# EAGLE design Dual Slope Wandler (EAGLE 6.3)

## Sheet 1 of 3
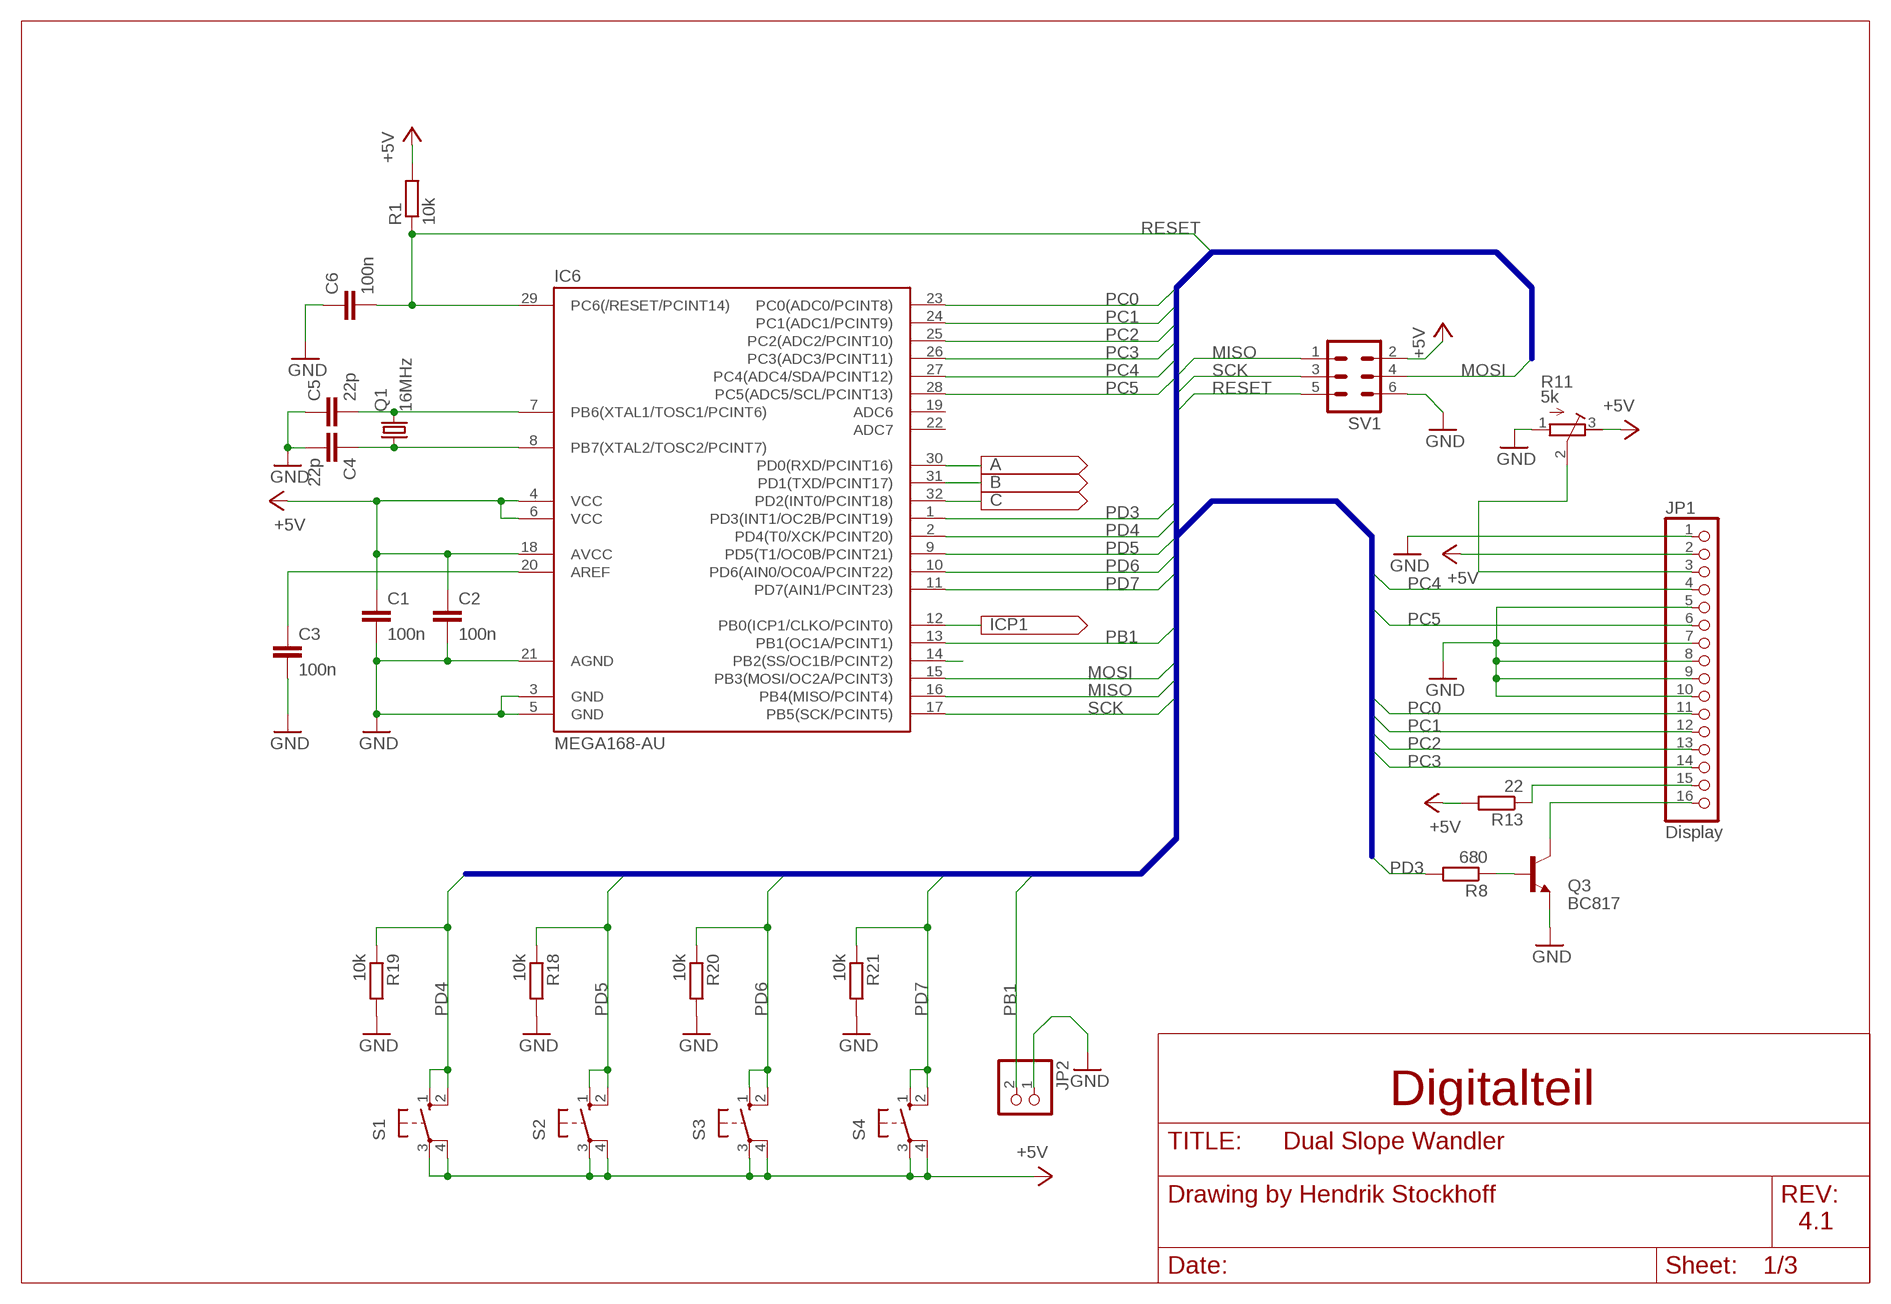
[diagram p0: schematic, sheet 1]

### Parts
C1  100n  C-EUC0805  [C0805]
C2  100n  C-EUC0805  [C0805]
C3  100n  C-EUC0805  [C0805]
C4  22p  C-EUC0805  [C0805]
C5  22p  C-EUC0805  [C0805]
C6  100n  C-EUC0805  [C0805]
IC6  MEGA168-AU  MEGA48/88/168-AU  [TQFP32-08]
JP1  Display  PINHD-1X16  [1X16]
JP2  PINHD-1X2  [1X02]
Q1  16MHz  CRYSTAL  [MT]
Q3  BC817  BC817-40SMD  [SOT23-BEC]
R1  10k  R-EU_R0805  [R0805]
R8  680  R-EU_R0805  [R0805]
R11  5k  R-TRIMM  [RTRIMC33X-2]
R13  22  R-EU_R0805  [R0805]
R18  10k  R-EU_R0805  [R0805]
R19  10k  R-EU_R0805  [R0805]
R20  10k  R-EU_R0805  [R0805]
R21  10k  R-EU_R0805  [R0805]
S1  10-XX  [B3F-10XX]
S2  10-XX  [B3F-10XX]
S3  10-XX  [B3F-10XX]
S4  10-XX  [B3F-10XX]
SV1  ML6  [ML6]

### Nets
+5V: C1.1 C2.1 IC6.4(VCC) IC6.6(VCC) IC6.18(AVCC) JP1.2 R1.2 R11.3(A) R13.2 S1.3(P) S1.4(P1) S2.3(P) S2.4(P1) S3.3(P) S3.4(P1) S4.3(P) S4.4(P1) SV1.2 ; also sheet 2,3
A: IC6.30(PD0(RXD/PCINT16)) ; also sheet 2
B: IC6.31(PD1(TXD/PCINT17)) ; also sheet 2
C: IC6.32(PD2(INT0/PCINT18)) ; also sheet 2
GND: C1.2 C2.2 C3.2 C4.2 C5.1 C6.1 IC6.3(GND) IC6.5(GND) IC6.21(AGND) JP1.1 JP1.5 JP1.7 JP1.8 JP1.9 JP1.10 JP2.1 Q3.E R11.1(E) R18.2 R19.2 R20.2 R21.2 SV1.6 ; also sheet 2,3
MISO: IC6.16(PB4(MISO/PCINT4)) SV1.1
MOSI: IC6.15(PB3(MOSI/OC2A/PCINT3)) SV1.4
N$4: JP1.3 R11.2(S)
N$6: C4.1 IC6.8(PB7(XTAL2/TOSC2/PCINT7)) Q1.1
N$7: C5.2 IC6.7(PB6(XTAL1/TOSC1/PCINT6)) Q1.3
N$15: IC6.14(PB2(SS/OC1B/PCINT2))
N$22: C3.1 IC6.20(AREF)
N$23: JP1.16 Q3.C
N$24: Q3.B R8.1
N$25: JP1.15 R13.1
PB0: IC6.12(PB0(ICP1/CLKO/PCINT0)) ; also sheet 2
PB1: IC6.13(PB1(OC1A/PCINT1)) JP2.2
PC0: IC6.23(PC0(ADC0/PCINT8)) JP1.11
PC1: IC6.24(PC1(ADC1/PCINT9)) JP1.12
PC2: IC6.25(PC2(ADC2/PCINT10)) JP1.13
PC3: IC6.26(PC3(ADC3/PCINT11)) JP1.14
PC4: IC6.27(PC4(ADC4/SDA/PCINT12)) JP1.4
PC5: IC6.28(PC5(ADC5/SCL/PCINT13)) JP1.6
PD3: IC6.1(PD3(INT1/OC2B/PCINT19)) R8.2
PD4: IC6.2(PD4(T0/XCK/PCINT20)) R19.1 S1.1(S) S1.2(S1)
PD5: IC6.9(PD5(T1/OC0B/PCINT21)) R18.1 S2.1(S) S2.2(S1)
PD6: IC6.10(PD6(AIN0/OC0A/PCINT22)) R20.1 S3.1(S) S3.2(S1)
PD7: IC6.11(PD7(AIN1/PCINT23)) R21.1 S4.1(S) S4.2(S1)
RESET: C6.2 IC6.29(PC6(/RESET/PCINT14)) R1.1 SV1.5
SCK: IC6.17(PB5(SCK/PCINT5)) SV1.3
Unconnected: IC6.19(ADC6) IC6.22(ADC7)

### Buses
MISO,MOSI,SCK,RESET,PC[0..5],PD[0..7],PB1

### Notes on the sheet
- Digitalteil
- 4.1

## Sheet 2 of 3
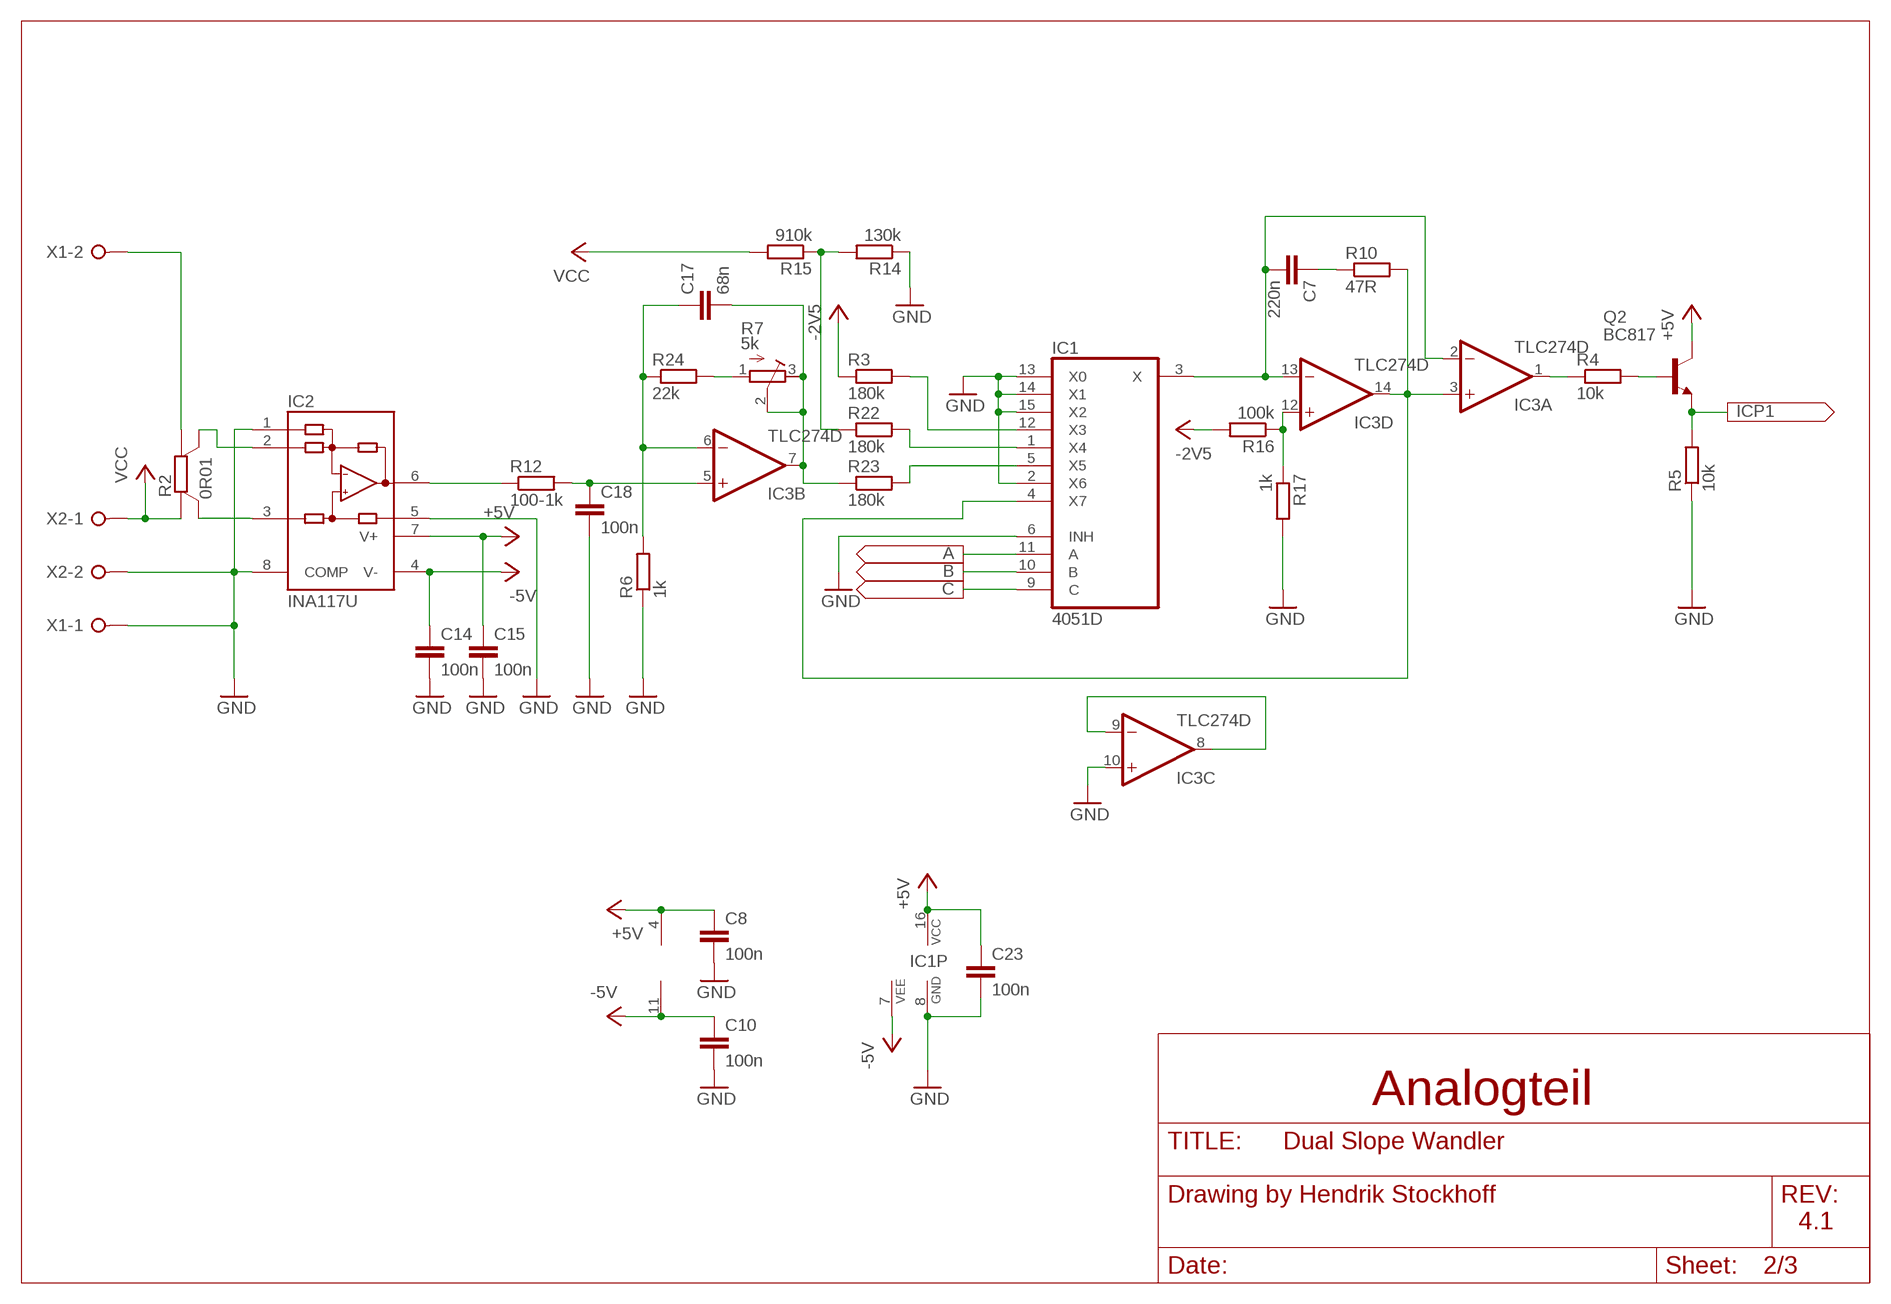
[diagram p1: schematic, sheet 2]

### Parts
C7  220n  C5/3  [C5B3]
C8  100n  C-EUC0805  [C0805]
C10  100n  C-EUC0805  [C0805]
C14  100n  C-EUC0805  [C0805]
C15  100n  C-EUC0805  [C0805]
C17  68n  C-EUC1206  [C1206]
C18  100n  C-EUC1206  [C1206]
C23  100n  C-EUC0805  [C0805]
IC1  4051D  [SO16]
IC2  INA117U  [SO08]
IC3  TLC274D  [SO14]
Q2  BC817  BC817-40SMD  [SOT23-BEC]
R2  0R01  PBV  [PBV]
R3  180k  R-EU_R0805  [R0805]
R4  10k  R-EU_R1206  [R1206]
R5  10k  R-EU_R1206  [R1206]
R6  1k  R-EU_R0805  [R0805]
R7  5k  R-TRIMM  [RTRIMC33X-2]
R10  47R  R-EU_R0805  [R0805]
R12  100-1k  R-EU_R0805  [R0805]
R14  130k  R-EU_R1206  [R1206]
R15  910k  R-EU_R1206  [R1206]
R16  100k  R-EU_R1206  [R1206]
R17  1k  R-EU_R1206  [R1206]
R22  180k  R-EU_R1206  [R1206]
R23  180k  R-EU_R0805  [R0805]
R24  22k  R-EU_R0805  [R0805]
X1  W237-02P  [W237-132]
X2  W237-02P  [W237-132]

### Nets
+5V: C8.1 C15.1 C23.1 IC1.16(VCC) IC2.7(V+) IC3.4(P:V+) Q2.C ; also sheet 1,3
-2V5: R3.1 R16.2 ; also sheet 3
-5V: C10.1 C14.1 IC1.7(VEE) IC2.4(V-) IC3.11(P:V-) ; also sheet 3
A: IC1.11(A) ; also sheet 1
B: IC1.10(B) ; also sheet 1
C: IC1.9(C) ; also sheet 1
GND: C8.2 C10.2 C14.2 C15.2 C18.2 C23.2 IC1.2(X6) IC1.6(INH) IC1.8(GND) IC1.13(X0) IC1.14(X1) IC1.15(X2) IC2.1(REFB) IC2.5(REFA) IC2.8(COMP) IC3.10(C:+IN) R5.1 R6.1 R14.1 R17.2 X1.1 X2.2 ; also sheet 1,3
N$5: C7.1 R10.1
N$8: IC2.6(OUT) R12.1
N$9: R2.I1(A) X1.2
N$10: IC1.4(X7) IC3.3(A:+IN) IC3.14(D:OUT) R10.2
N$11: IC3.8(C:OUT) IC3.9(C:-IN)
N$12: IC3.1(A:OUT) R4.1
N$13: Q2.B R4.2
N$14: IC1.5(X5) R23.2
N$16: R14.2 R15.1 R22.1
N$17: IC2.3(+IN) R2.U2(SB)
N$18: C18.1 IC3.5(B:+IN) R12.2
N$20: IC2.2(-IN) R2.U1(SA)
N$26: C17.2 IC3.7(B:OUT) R7.2(S) R7.3(A) R23.1
N$27: IC3.12(D:+IN) R16.1 R17.1
N$28: IC1.1(X4) R22.2
N$29: IC1.12(X3) R3.2
N$30: C7.2 IC1.3(X) IC3.2(A:-IN) IC3.13(D:-IN)
N$33: C17.1 IC3.6(B:-IN) R6.2 R24.1
N$35: R7.1(E) R24.2
PB0: Q2.E R5.2 ; also sheet 1
VCC: R2.I2(B) R15.2 X2.1 ; also sheet 3

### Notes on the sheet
- Analogteil
- 4.1

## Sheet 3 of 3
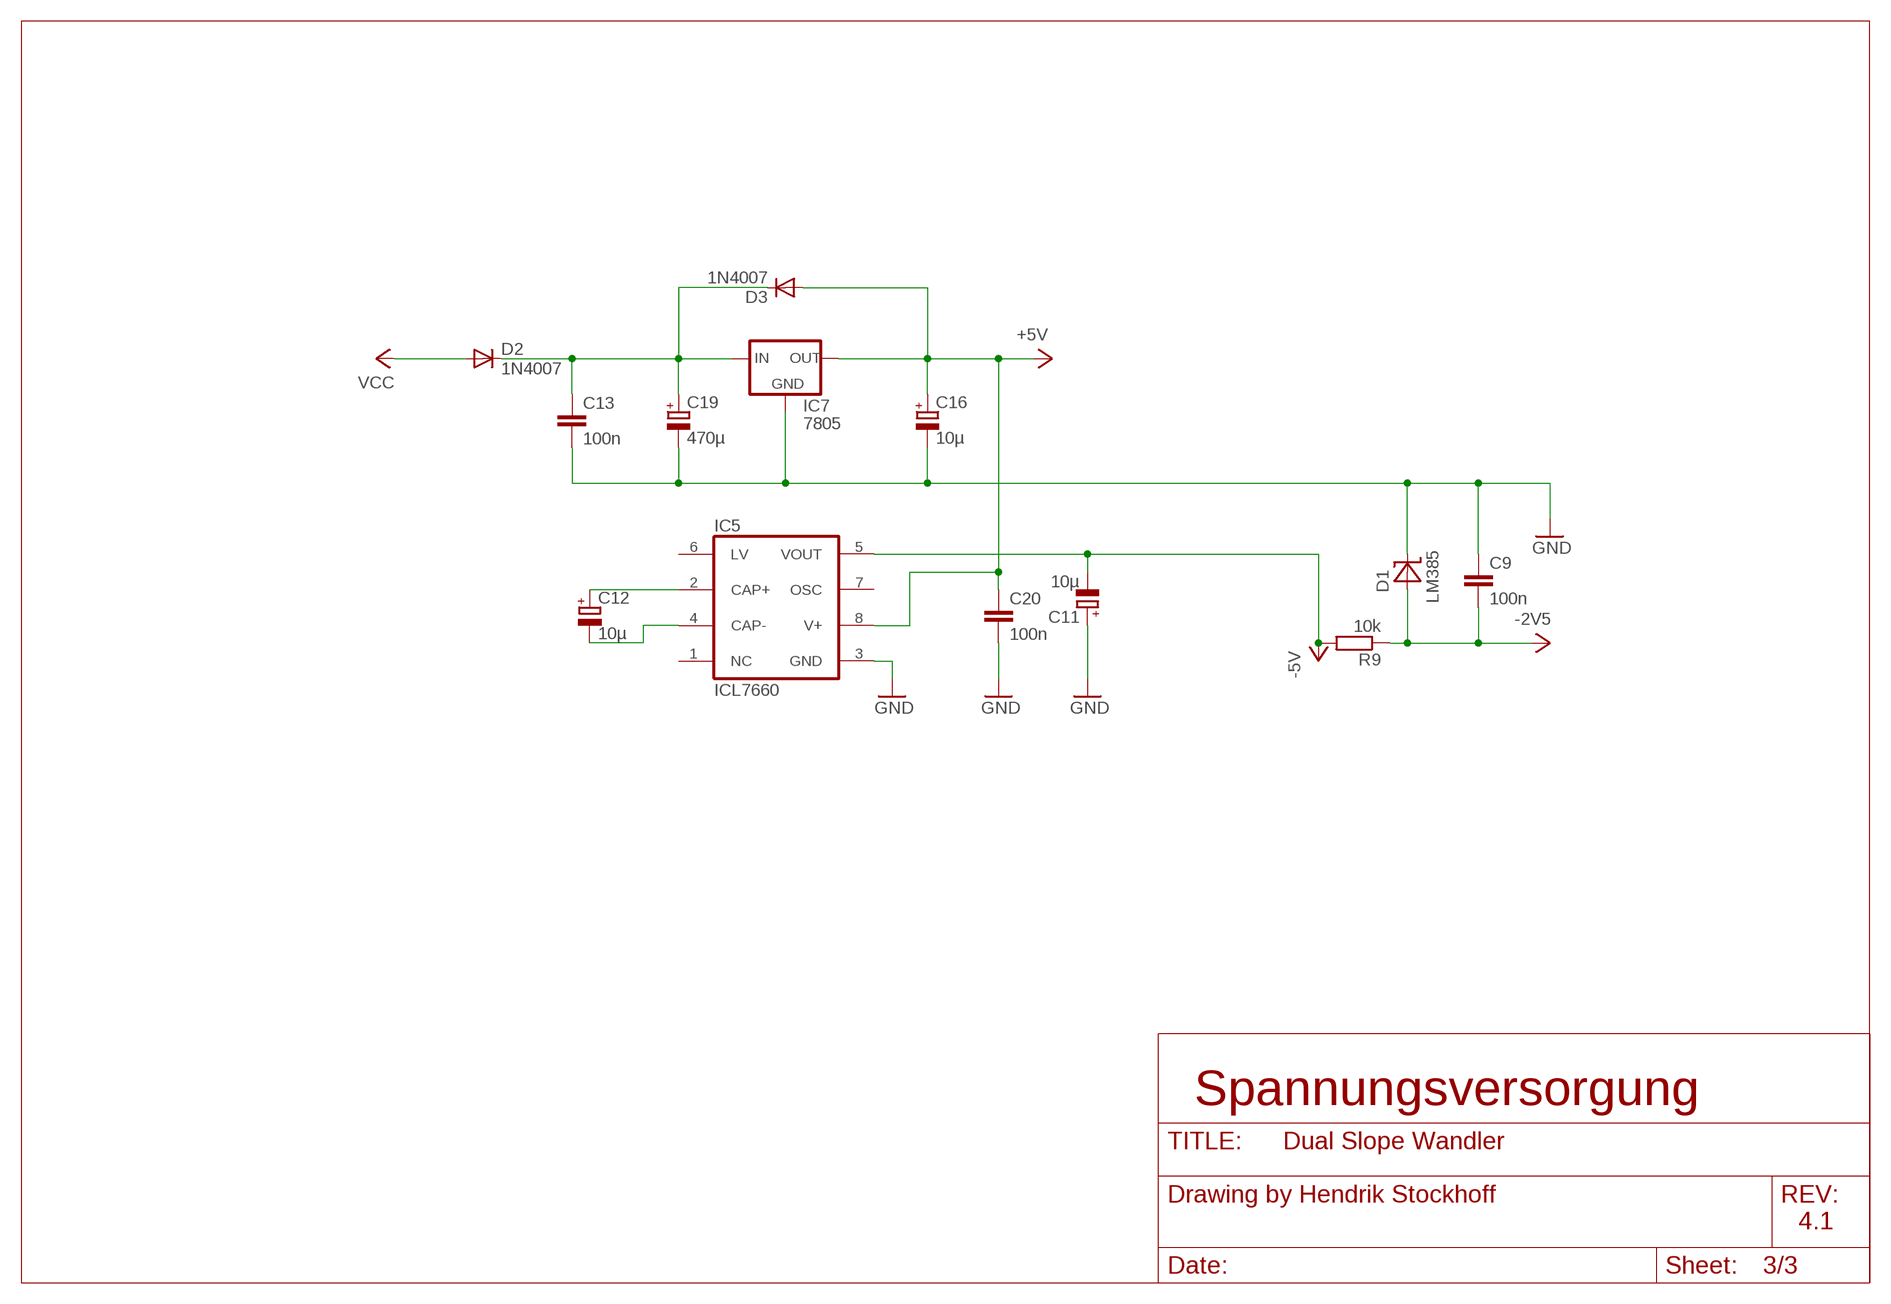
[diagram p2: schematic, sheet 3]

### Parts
C9  100n  C-EUC0805  [C0805]
C11  10µ  CPOL-EUE2-5  [E2-5]
C12  10µ  CPOL-EUE2-5  [E2-5]
C13  100n  C5/3  [C5B3]
C16  10µ  CPOL-EUE2-5  [E2-5]
C19  470µ  CPOL-EUE5-10.5  [E5-10,5]
C20  100n  C5/3  [C5B3]
D1  LM385  LM385M3-2,5  [SOT23]
D2  1N4007  DIODE-MELF-MLL41  [MELF-MLL41]
D3  1N4007  DIODE-MELF-MLL41  [MELF-MLL41]
IC5  ICL7660  ICL7660CSA  [SO08]
IC7  7805  78XXS  [78XXS]
R9  10k  R-EU_R0805  [R0805]

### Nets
+5V: C16.+ C20.1 D3.A IC5.8(V+) IC7.OUT ; also sheet 1,2
-2V5: C9.2 D1.2(-) R9.1 ; also sheet 2
-5V: C11.- IC5.5(VOUT) R9.2 ; also sheet 2
GND: C9.1 C11.+ C13.2 C16.- C19.- C20.2 D1.1(+) IC5.3(GND) IC7.GND ; also sheet 1,2
N$2: C12.+ IC5.2(CAP+)
N$3: C12.- IC5.4(CAP-)
N$45: C13.1 C19.+ D2.C D3.C IC7.IN
VCC: D2.A ; also sheet 2
Unconnected: IC5.1(NC) IC5.6(LV) IC5.7(OSC)

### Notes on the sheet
- Spannungsversorgung
- 4.1

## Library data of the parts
C1-C6 C8-C10 C14 C15 C17 C18 C23 = rcl:C-EU: CAPACITOR, European symbol
C7 C13 C20 = capacitor-wima:C: CAPACITOR
C11 C12 C16 C19 = rcl:CPOL-EU: POLARIZED CAPACITOR, European symbol
D1 = texas:LM385M3-2,5
D2 D3 = diode:DIODE-: DIODE
IC1 = 40xx:4051: 8-channel ANALOG MULTIPLEXER
IC2 = burr-brown:INA117: Difference Amplifier High Common-Mode Voltage; MF: TEXAS INSTRUMENTS; MPN: INA117KU; OC_FARNELL: 1706653; OC_NEWARK: 17M6717
IC3 = linear:TLC274: OP AMP
IC5 = maxim:ICL7660CSA: VOLTAGE CONVERTER; MF: MAXIM; MPN: ICL7660CSA; OC_FARNELL: 9724710; OC_NEWARK: 34C3732
IC6 = avr-7:MEGA48/88/168
IC7 = v-reg:78XXS: VOLTAGE REGULATOR
JP1 = pinhead:PINHD-1X16: PIN HEADER
JP2 = pinhead:PINHD-1X2: PIN HEADER
Q1 = crystal:CRYSTAL
Q2 Q3 = transistor-npn:BC817*: NPN Transistor
R1 R3-R6 R8-R10 R12-R24 = rcl:R-EU_: RESISTOR, European symbol
R2 = resistor-shunt:PBV: Isabellenhütte PBV resistor
R7 R11 = rcl:R-TRIMM: Trimm resistor
S1-S4 = switch-omron:10-XX: OMRON SWITCH; MPN: B3F-1000; OC_FARNELL: 176432; OC_NEWARK: 36M3542
SV1 = con-harting-ml:ML6: HARTING; OC_FARNELL: unknown; OC_NEWARK: unknown
X1 X2 = con-wago-508:W237-02P: WAGO SREW CLAMP; OC_FARNELL: unknown; OC_NEWARK: unknown

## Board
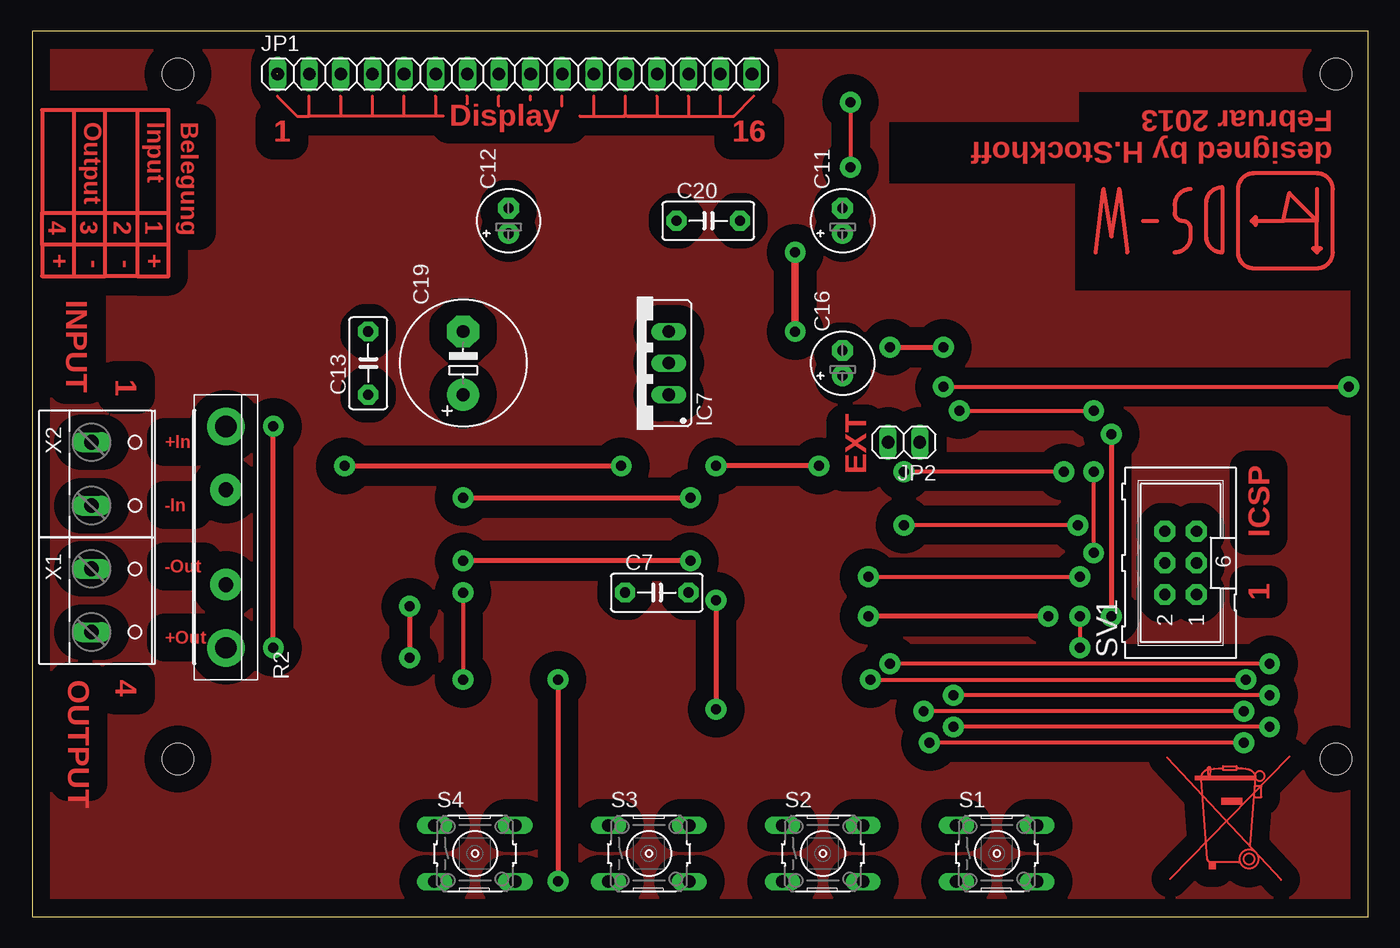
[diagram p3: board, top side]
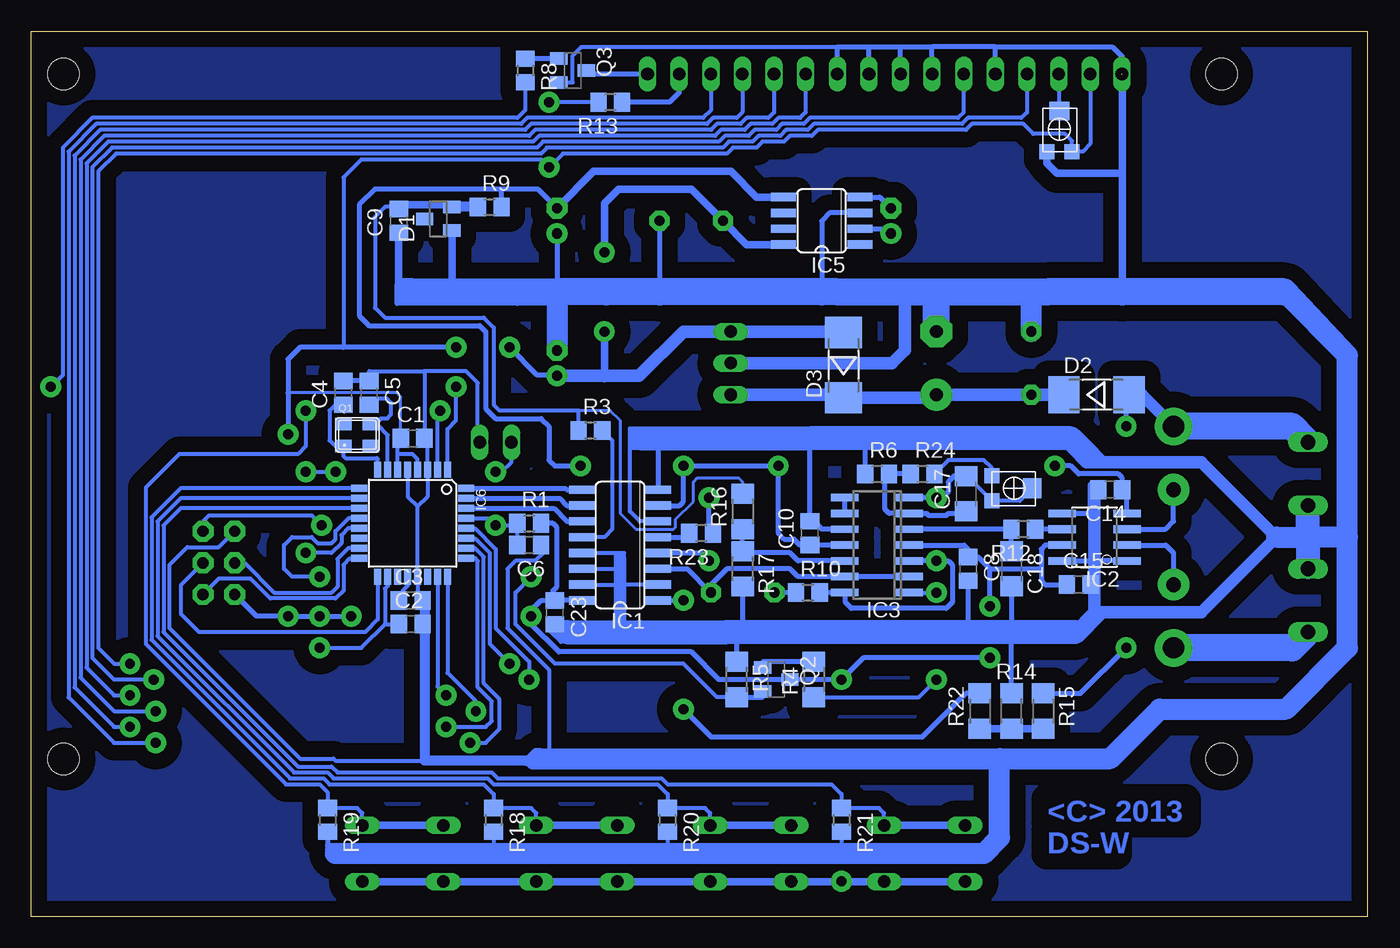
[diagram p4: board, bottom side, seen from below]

Size 107.31 x 71.11 mm. Coordinates in mm from the lower left corner, seen from the top.
Outline: 0,0 107.32,0 107.32,12.38 107.3,71.11 0,71.11 0,0
Copper layers (1*16): Top 0.035mm / dielectric 1.5mm / Bottom 0.035mm
Design rules: minimum track width 6mil, minimum drill 0.3mm, track to track 6mil, track to pad 6mil, pad to pad 6mil, via to via 6mil, smd to smd 6mil, copper to edge 20mil, drill to drill 10mil, minimum pad ring 8mil, minimum via ring 6mil, stop-mask expansion 3mil, vias tented up to drill 0mil, thermal gap 8mil
Holes 2.5 mm at 11.71,12.66 104.71,12.66 11.71,67.66 104.71,67.66

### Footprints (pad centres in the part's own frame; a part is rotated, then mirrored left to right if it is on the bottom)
C0805 = smd 1.3 x 1.5: 1 -0.95,0; 2 0.95,0
C5B3 = drill 0.813 pad 1.6 octagon: 1 -2.54,0; 2 2.54,0
E2-5 = drill 0.813 pad 1.676: + -1.016,0 | drill 0.813 pad 1.676 octagon: - 1.016,0
C1206 = smd 1.6 x 1.8: 1 -1.4,0; 2 1.4,0
E5-10,5 = drill 1.016 pad 2.54: + -2.54,0 | drill 1.016 pad 2.54 octagon: - 2.54,0
SOT23 = smd 1 x 1.4: 1 -0.95,-1.1; 2 0.95,-1.1; 3 0,1.1
MELF-MLL41 = smd 2.5 x 3: A 2.625,0; C -2.625,0
SO16 = smd 0.66 x 2.032: 1 -4.445,-3.073; 2 -3.175,-3.073; 3 -1.905,-3.073; 4 -0.635,-3.073; 5 0.635,-3.073; 6 1.905,-3.073; 7 3.175,-3.073; 8 4.445,-3.073; 9 4.445,3.073; 10 3.175,3.073; 11 1.905,3.073; 12 0.635,3.073; 13 -0.635,3.073; 14 -1.905,3.073; 15 -3.175,3.073; 16 -4.445,3.073
SO08 = smd 0.61 x 2.21: 1 -1.905,-2.616; 2 -0.635,-2.616; 3 0.635,-2.616; 4 1.905,-2.616; 5 1.905,2.616; 6 0.635,2.616; 7 -0.635,2.616; 8 -1.905,2.616
SO14 = smd 0.6 x 2.2: 1 -3.81,-2.6; 2 -2.54,-2.6; 3 -1.27,-2.6; 4 0,-2.6; 5 1.27,-2.6; 6 2.54,-2.6; 7 3.81,-2.6; 8 3.81,2.6; 9 2.54,2.6; 10 1.27,2.6; 11 0,2.6; 12 -1.27,2.6; 13 -2.54,2.6; 14 -3.81,2.6
SO08' = smd 0.66 x 2.032: 1 -1.905,-3.073; 2 -0.635,-3.073; 3 0.635,-3.073; 4 1.905,-3.073; 5 1.905,3.073; 6 0.635,3.073; 7 -0.635,3.073; 8 -1.905,3.073
TQFP32-08 = smd 1.27 x 0.559: 1 -4.293,2.8; 2 -4.293,2; 3 -4.293,1.2; 4 -4.293,0.4; 5 -4.293,-0.4; 6 -4.293,-1.2; 7 -4.293,-2; 8 -4.293,-2.8; 17 4.293,-2.8; 18 4.293,-2; 19 4.293,-1.2; 20 4.293,-0.4; 21 4.293,0.4; 22 4.293,1.2; 23 4.293,2; 24 4.293,2.8 | smd 0.559 x 1.27: 9 -2.8,-4.293; 10 -2,-4.293; 11 -1.2,-4.293; 12 -0.4,-4.293; 13 0.4,-4.293; 14 1.2,-4.293; 15 2,-4.293; 16 2.8,-4.293; 25 2.8,4.293; 26 2,4.293; 27 1.2,4.293; 28 0.4,4.293; 29 -0.4,4.293; 30 -1.2,4.293; 31 -2,4.293; 32 -2.8,4.293
78XXS = drill 1.016 long: GND 0,-2.54; IN -2.54,-2.54; OUT 2.54,-2.54
1X16 = drill 1.016 long: 1 -19.05,0; 2 -16.51,0; 3 -13.97,0; 4 -11.43,0; 5 -8.89,0; 6 -6.35,0; 7 -3.81,0; 8 -1.27,0; 9 1.27,0; 10 3.81,0; 11 6.35,0; 12 8.89,0; 13 11.43,0; 14 13.97,0; 15 16.51,0; 16 19.05,0
1X02 = drill 1.016 long: 1 -1.27,0; 2 1.27,0
MT = smd 1.3 x 1: 1 0,0; 2 2.2,0; 3 2.2,1.8; 4 0,1.8
SOT23-BEC = smd 1 x 1.4: B -0.95,-1.1; C 0,1.1; E 0.95,-1.1
R0805 = smd 1.3 x 1.5: 1 -0.95,0; 2 0.95,0
PBV = drill 1.7 pad 3: I1 -8.89,0; I2 8.89,0 | drill 1.2 pad 2.54: U1 -3.81,0; U2 3.81,0
R1206 = smd 1.6 x 1.803: 1 -1.422,0; 2 1.422,0
RTRIMC33X-2 = smd 1.2 x 1.2: 1 -0.953,-1.746; 3 1.048,-1.746 | smd 1.6 x 1.5: 2 0.048,1.504
B3F-10XX = drill 1.016 long: 1 -3.251,2.261; 2 3.251,2.261; 3 -3.251,-2.261; 4 3.251,-2.261
ML6 = drill 0.914 pad 1.676 octagon: 1 -2.54,-1.27; 2 -2.54,1.27; 3 0,-1.27; 4 0,1.27; 5 2.54,-1.27; 6 2.54,1.27
W237-132 = drill 1.194 long: 1 -2.54,-0.635; 2 2.54,-0.635

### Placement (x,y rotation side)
C1  76.68,38.42 0 bottom
C2  76.83,23.5 0 bottom
C3  76.83,25.4 0 bottom
C4  82.23,42.07 90 bottom
C5  80.17,42.07 270 bottom
C6  67.31,29.84 180 bottom
C7  50.17,26.04 0 top
C8  32.07,27.94 270 bottom
C9  77.79,55.88 90 bottom
C10  44.77,30.8 90 bottom
C11  65.09,55.88 90 top
C12  38.26,55.88 90 top
C13  26.99,44.45 90 top
C14  20.64,34.29 180 bottom
C15  23.18,26.67 0 bottom
C16  65.09,44.45 90 top
C17  32.23,33.97 90 bottom
C18  28.57,27.94 270 bottom
C19  34.61,44.45 90 top
C20  54.29,55.88 0 top
C23  65.25,24.45 270 bottom
D1  74.61,56.04 90 bottom
D2  21.75,41.91 0 bottom
D3  42.07,44.29 90 bottom
IC1  60.01,29.84 90 bottom
IC2  21.91,30.48 90 bottom
IC3  39.37,29.84 90 bottom
IC5  ICL7660  [SO08']  43.81,55.88 90 bottom
IC6  76.68,31.59 270 bottom
IC7  48.58,44.45 90 top
JP1  38.76,67.66 0 top
JP2  70.01,38.1 180 top
Q1  82.23,37.78 0 bottom
Q2  47.47,19.05 270 bottom
Q3  63.82,67.94 270 bottom
R1  67.31,31.59 0 bottom
R2  15.56,30.48 90 top
R3  62.39,39.05 0 bottom
R4  44.45,19.05 90 bottom
R5  50.64,19.05 270 bottom
R6  39.37,35.56 0 bottom
R7  28.42,34.45 270 bottom
R8  67.63,67.94 270 bottom
R9  70.48,56.99 0 bottom
R10  44.93,26.04 0 bottom
R11  24.77,63.18 0 bottom
R12  27.62,31.11 180 bottom
R13  60.8,65.41 180 bottom
R14  28.57,16.51 270 bottom
R15  26.04,16.51 90 bottom
R16  50.17,32.54 90 bottom
R17  50.17,27.94 270 bottom
R18  70.17,7.78 270 bottom
R19  83.5,7.78 270 bottom
R20  56.2,7.78 270 bottom
R21  42.23,7.78 270 bottom
R22  31.11,16.51 90 bottom
R23  53.5,30.8 180 bottom
R24  35.72,35.56 0 bottom
S1  77.47,5.08 0 top
S2  63.5,5.08 0 top
S3  49.53,5.08 0 top
S4  35.56,5.08 0 top
SV1  92.23,28.42 90 top
U$2  [MULLTONNE_TOP]  90.49,2.54 0 top
X1  5.4,25.4 270 top
X2  5.4,35.56 270 top

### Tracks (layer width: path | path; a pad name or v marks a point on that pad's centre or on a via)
+5V  (via drill 0.8 pad 1.68)
  Top 0.305: v65.72,65.41 v65.72,60.17 | v84.14,24.13 v84.14,21.59
  Top 0.406: v81.6,24.13 v67.15,24.13 | v30.32,24.92 v30.32,20.8 | v42.23,19.05 v42.23,2.86 | v68.9,45.72 v73.18,45.72 | v86.68,38.73 v86.68,24.13
  Top 0.61: v61.28,53.34 v61.28,46.99
  Bottom 0.254: v42.23,2.86 42.23,2.82 | C16.+ 65.09,43.5 | 82.23,45.88 82.23,45.72 | C1.1 77.63,41.75 77.95,42.07 86.68,42.07
  Bottom 0.305: 77.88,37.15 IC6.6 77.88,38.33 77.79,38.42 | 77.88,37.15 77.88,37.69 C1.1 | IC6.4 76.28,36.75 76.68,37.15 77.88,37.15 | IC6.18 78.68,26.57 78.9,26.35 78.9,23.5 | 78.9,23.5 C2.1 | R13.2 v65.72,65.41 | 82.23,45.88 82.23,59.37 80.8,60.8 66.36,60.8 v65.72,60.17 64.61,61.28 51.43,61.28 50.96,61.75 49.05,61.75 48.58,62.23 46.83,62.23 46.36,62.71 44.61,62.71 44.13,63.18 32.23,63.18 31.75,63.66 27.62,63.66 26.83,62.86 24.29,62.86 23.72,62.29 R11.3 22.86,61.44 22.25,62.05 JP1.2 | v84.14,21.59 80.8,21.59 78.9,23.5 | 65.4,25.4 C23.1
  Bottom 0.406: IC2.7 25.88,29.84 26.19,29.53 26.19,27.94 | 26.19,27.94 26.19,26.99 25.88,26.67 C15.1 | IC3.4 32.38,29.84 32.07,29.53 C8.1 31.27,28.89 30.32,27.94 | IC1.16 65.4,25.4 | 65.4,25.4 C23.1 | v81.6,24.13 v84.14,24.13 v86.68,24.13 89.22,24.13 SV1.2 | 65.4,25.4 66.36,25.4 67.15,24.61 v67.15,24.13 67.15,23.5 64.93,21.27 54.29,21.27 52.07,19.05 Q2.C v42.23,19.05 40.48,20.8 v30.32,20.8 | 65.4,25.4 65.4,26.2 65.09,26.51 65.09,31.27 65.4,31.59 R1.2 | 30.32,27.94 26.19,27.94 | v30.32,24.92 30.32,27.94 | 65.09,43.5 66.68,43.5 v68.9,45.72 | v73.18,45.72 82.23,45.72 85.72,45.72 86.68,44.77 86.68,42.07 v86.68,38.73
  Bottom 0.61: S4.3 S4.4 | S4.4 42.23,2.82 S3.3 S3.4 S2.3 | S2.3 60.45,2.82 | S2.3 S2.4 S1.3 S1.4 | S4.4 32.26,2.82 32.23,2.86 32.23,3.02 | v61.28,53.34 61.28,57.28 60.13,58.42 54.29,58.42 C20.1 49.85,53.97 IC5.8 | v61.28,46.99 61.28,43.18 C16.+
  Bottom 1.016: D3.A 42.07,46.99 IC7.OUT 54.93,46.99 58.48,43.43 C16.+
-2V5
  Bottom 0.254: 63.34,40.64 60.8,40.64 60.01,39.85 60.01,32.39 58.74,31.11 55.72,31.11 55.56,31.27 55.56,31.91 54.13,33.34 54.13,34.92 53.82,35.24 50.48,35.24 50.17,34.92 R16.2
  Bottom 0.305: R3.1 63.34,40.64 63.66,40.64 69.69,40.64 70.17,41.12 70.17,47.31 70.96,48.1 78.9,48.1 79.69,48.89 79.69,56.2 78.9,56.99 D1.2
  Bottom 0.61: D1.2 73.66,56.99 73.82,57.15 77.47,57.15 C9.2
  Bottom 0.813: R9.1 D1.2
-5V  (via drill 0.8 pad 1.68)
  Top 0.406: v25.08,36.2 v47.31,36.2 | v63.18,36.2 v54.93,36.2
  Bottom 0.406: IC3.11 44.58,29.84 C10.1 45.56,29.84 46.04,30.32 46.83,30.32 47.31,30.8 v47.31,36.2 v54.93,36.2 54.93,33.34 55.25,33.02 IC1.7 | IC2.4 19.29,33.89 C14.1 19.69,35.25 20,35.56 23.18,35.56 23.81,36.2 v25.08,36.2 | 69.69,58.42 66.61,58.42 C11.- | 69.69,58.42 79.69,58.42 80.96,57.15 80.96,48.26 80.17,47.47 71.28,47.47 70.8,46.99 70.8,40.8 70.01,40 66.36,40 65.72,39.37 65.72,36.67 65.25,36.2 v63.18,36.2 | R9.2 69.54,58.26 69.69,58.42
  Bottom 0.61: IC5.5 49.05,57.78 51.12,59.85 62.13,59.85 C11.-
A
  Bottom 0.406: IC6.30 65.33,32.79 64.29,31.75 IC1.11
B
  Bottom 0.406: IC6.31 64.86,33.59 64.29,33.02 IC1.10
C
  Bottom 0.406: IC6.32 64.4,34.39 64.29,34.29 IC1.9
GND  (1 unrouted)
  Bottom 0.254: 59.21,39.21 58.26,39.21 58.26,38.58 59.05,38.58
  Bottom 0.305: IC1.6 58.42,31.75 59.21,32.54 59.21,39.21 | IC6.5 77.08,33.74 77.07,33.74 76.28,32.94 | IC6.21 76.28,32.94 | 76.28,32.94 75.48,33.74 IC6.3 75.48,38.17 C1.2 75.72,43.81 | IC6.21 76.28,25.48 C3.2 C2.2 | R18.2 70.17,5.08 70.01,5.08 | R20.2 56.2,5.08 56.04,5.08 | R21.2 42.23,5.08 | C6.1 66.2,29.52 | IC6.21 76.28,25.95 75.72,25.4 | 75.72,12.54 82.87,12.54 83.03,12.7 85.72,12.7 96.2,23.18 96.2,28.26 94.77,29.69 92.23,29.69 SV1.6 | 76.68,51.12 77.79,51.12 | Q3.E 63.82,66.99 63.82,69.14 63.11,69.85 42.23,69.85 | 25.77,50.17 25.72,50.17 | 21.91,34.77 22.23,34.77 | 68.26,49.21 77.95,49.21 77.95,50.8 77.79,50.8 77.79,49.37 | 57.31,39.05 57.31,39.21 57.63,39.21 | 59.21,39.21 57.63,39.21 | 57.31,39.05 57.63,39.21 | 59.05,37.78 59.05,37.62 57.47,37.62 56.93,38.1 | 57.31,39.05 57.47,38.42 | 66.2,29.52 66.2,29.69 | 66.52,12.7 66.36,13.02 65.72,13.18 65.72,19.84 69.06,23.18 69.06,27.94 68.42,28.57 66.83,28.57 66.2,29.21 66.2,29.52 | C5.1 80.17,43.81 75.72,43.81 | 59.21,39.21 58.42,39.05 | 63.02,23.02 63.34,23.02 64.29,22.86 | JP2.1 71.44,38.1 71.44,42.86 72.39,43.81 75.72,43.81 | 63.82,22.07 64.77,22.07 65.56,22.86 65.25,22.86 | 65.25,22.86 65.09,22.7 61.91,22.7 | 65.25,22.86 C23.2 | 58.74,23.18 60.01,23.18 | 60.17,28.89 60.09,28.81 | 60.09,28.81 60.01,28.73 | IC1.15 60.01,26.67 IC1.2 | IC1.14 60.01,27.94 60.01,27.78 | IC1.13 60.32,29.21 | 60.32,29.21 59.69,29.21 59.69,28.81 60.09,28.81 | 60.32,28.73 60.32,29.21
  Bottom 0.34: 23.65,23.65 23.18,23.65 23.18,23.34
  Bottom 0.406: IC2.8 21.91,28.57 IC2.1 21.59,28.57 21.91,28.89 | 21.91,27.3 21.91,26.67 | IC2.5 21.91,32.39 | R6.1 40.32,36.83 40.32,38.42 | C8.2 32.07,22.86 | IC3.10 43.82,31.11 44.77,32.07 | 44.77,32.07 44.61,32.04 C10.2 44.77,32.07 | 44.77,32.07 44.77,38.42 | R14.1 28.57,22.86 C18.2 | R5.1 50.64,22.86 | R17.2 50.17,22.86 | 51.43,22.86 51.12,22.86 | 58.74,23.18 58.42,22.86 | IC1.8 56.93,38.1 56.93,38.2 56.83,38.42 | 21.91,34.45 C14.2 21.91,34.29 21.91,34.45 | 29.87,69.85 JP1.5 29.87,69.71 30,69.85 | 29.87,69.85 30,69.85 | 30,69.85 34.95,69.85 | JP1.7 34.95,69.85 | JP1.8 37.49,69.85 | 37.49,69.85 34.95,69.85 | JP1.9 40.03,69.85 | 40.03,69.85 37.49,69.85 | JP1.10 42.57,69.85 42.23,69.85 40.03,69.85 | C5.1 C4.2 | 29.87,69.85 20.48,69.85 19.68,69.06 19.68,67.68 | 1.27,45.4 1.59,45.4 1.59,45.08 | 22.23,32.86 22.23,34.77 | 21.91,34.45 21.91,34.77 | 65.72,13.18 66.68,13.34 66.83,13.34 | 66.83,13.34 67.63,12.54 67.15,12.06 66.36,12.06 | 66.83,13.34 66.36,13.02 | 66.2,12.06 66.36,12.06 | 66.36,12.06 66.52,12.22 66.83,12.22 | C20.2 56.83,50.17 | IC5.3 43.18,56.52 43.82,55.88 43.82,50.17 | C11.+ 65.09,50.32 60.96,50.32 | 19.68,67.63 19.71,67.63 JP1.1 | 63.34,23.02 65.25,23.02 C23.2 | 59.05,39.05 59.05,38.58 59.05,38.1 | R19.2 83.5,5.71 | 83.5,5.71 83.5,5.4 | 83.5,5.4 83.5,4.92 | 82.87,5.08 83.19,5.08 83.5,5.4 | 81.91,5.71 83.5,5.71
  Bottom 0.61: D1.1 73.51,50.32 | 73.51,50.32 73.51,50.18 73.5,50.17 | 61.12,50.17 60.96,50.32 | C9.1 77.79,51.12 77.79,50.8 77.79,50.64 76.99,50.17 | 73.67,50.17 73.51,50.32 | 19.68,67.63 19.68,59.69 | 19.68,59.69 19.68,50.17 | R11.1 25.72,60.48 24.92,59.69 19.68,59.69
  Bottom 0.7: 22.8,23.34 22.7,23.5 | 23.18,23.34 22.8,23.34 | 22.8,23.34 23.15,23.21
  Bottom 0.813: 21.91,26.67 C15.2 | 75.72,25.4 75.72,12.54 67.63,12.54 66.83,12.54 66.52,12.7 | 6.19,50.64 1.27,45.4 | 4.76,32.86 X2.2 | X1.1 4.76,28.1
  Bottom 1.016: 21.91,28.57 21.91,27.3 21.91,26.67 | 21.91,26.67 21.91,24.45 | 21.91,24.45 13.34,24.45 7.3,30.48 13.34,36.51 21.27,36.51 | 21.91,36.51 21.27,36.51 | 21.91,24.45 23.49,22.86 23.65,22.86 23.81,22.7 23.31,22.7 23.23,22.79 | IC7.GND 38.16,44.45 37.15,45.47 37.15,50.01 42.54,50.17 | 21.91,28.89 21.91,32.39 21.91,34.45 | 21.91,36.51 22.78,37.39 | 23.02,38.26 21.27,36.51 | 21.91,36.51 22.54,36.51 | 22.38,36.67 22.54,36.51 | 22.54,36.51 23.65,37.62 | 21.43,24.29 23.18,22.54 23.23,22.79 | 23.23,22.79 23.15,23.21 23.34,23.18 | 60.01,23.18 60.01,26.67 60.01,27.78 | 60.01,27.94 60.01,28.73
  Bottom 1.27: 5.08,30.48 4.76,30.16
  Bottom 1.676: 7.3,30.48 5.08,30.48 | C13.2 26.99,50.17 | 60.96,50.32 65.09,50.17 C16.- | 82.87,5.08 70.01,5.08 56.04,5.08 42.23,5.08 30.8,5.08 29.53,6.35 29.53,12.7 | 29.53,12.7 20.64,12.7 16.67,16.67 6.51,16.67 1.59,21.59 1.59,30.48 | 1.59,30.48 4.76,30.48 | 1.59,30.48 1.59,45.08 6.67,50.17 | 66.52,12.7 29.53,12.7
  Bottom 1.93: 23.49,22.86 28.57,22.86 32.07,22.86 50.17,22.86 50.64,22.86 51.12,22.86 | 64.29,22.86 58.42,22.86 51.43,22.86 | 58.26,38.42 57.47,38.42 56.83,38.42 44.77,38.42 40.32,38.42 23.81,38.42 22.78,37.39 22.38,36.99 | 4.76,32.86 4.76,30.48 4.76,30.16 4.76,28.1
  Bottom 2.184: 34.61,50.17 26.99,50.17 25.72,50.17 19.68,50.17 6.67,50.17 | C19.- 34.61,50.17 | 34.61,50.17 42.54,50.17 43.82,50.17 56.83,50.17 61.12,50.17 65.09,50.17 73.5,50.17 | 76.99,50.17 73.67,50.17
MISO
  Bottom 0.305: 81.06,28.79 IC6.16 81.28,28.79 81.28,28.73 81.76,28.73 82.23,28.26 82.23,26.19 82.87,25.56 88.11,25.56 89.69,27.15 92.23,27.15 SV1.1
MOSI
  Bottom 0.305: IC6.15 81.85,29.59 82.71,28.73 82.71,26.51 83.19,26.04 87.79,26.04 90.17,28.42 SV1.4
N$1
  Top 0.305: 96.84,53.34 arc90 98.11,52.07 103.19,52.07 arc90 104.46,53.34 104.46,58.42 arc90 103.19,59.69 98.11,59.69 arc90 96.84,58.42 96.84,53.34
N$2
  Bottom 0.406: IC5.2 38.64,55.25 C12.+
N$3
  Bottom 0.406: IC5.4 39.15,57.78 C12.-
N$4
  Bottom 0.305: JP1.3 24.79,64.76 R11.2
N$5
  Bottom 0.406: R10.1 C7.1
N$6
  Bottom 0.305: IC6.8 79.48,36.77 79.53,36.83 82.07,36.83 82.23,36.99 Q1.1 82.87,37.78 83.34,38.26 83.34,40.64 82.87,41.12 C4.1
N$7
  Bottom 0.305: IC6.7 78.68,38.67 79.53,39.53 79.98,39.53 Q1.3 79.64,39.58 79.22,40 78.74,40 78.42,40.32 78.42,41.27 78.74,41.59 79.69,41.59 C5.2
N$8
  Bottom 0.406: IC2.6 R12.1
N$9
  Bottom 0.813: 5.08,22.54 X1.2
  Bottom 2.184: R2.I1 6.03,21.59 5.08,22.54
N$10  (via drill 0.8 pad 1.68)
  Top 0.406: v52.86,28.57 v34.61,28.57
  Bottom 0.406: R10.2 IC3.14 41.91,25.98 41.91,25.24 41.43,24.77 33.81,24.77 33.34,25.24 33.34,28.26 33.66,28.57 v34.61,28.57 IC3.3 | IC1.4 53.5,29.21 v52.86,28.57
N$11
  Bottom 0.406: IC3.9 IC3.8
N$12  (via drill 0.8 pad 1.68)
  Top 0.305: v34.61,26.04 v34.61,19.05
  Bottom 0.305: IC3.1 v34.61,26.04 | R4.1 36.03,17.63 v34.61,19.05
N$13
  Bottom 0.406: R4.2 48.57,20.47 Q2.B
N$14
  Bottom 0.406: IC1.5 54.77,30.48 54.61,30.64 R23.2
N$16
  Bottom 0.61: R15.1 R14.2 R22.1
N$17
  Bottom 0.406: IC2.3 16.19,31.11 15.56,31.75 R2.U2
N$18
  Bottom 0.406: R12.2 | R12.2 IC3.5 | C18.1 R12.2
N$19
  Top 0.305: 103.19,58.42 103.19,55.88 | 103.19,53.34 103.5,53.66 102.87,53.66 103.19,53.34 | 103.19,53.34 103.19,55.88 | 103.19,55.88 100.49,55.88 | 97.95,55.88 98.27,56.2 98.27,55.56 97.95,55.88 | 97.95,55.88 100.49,55.88 | 100.49,55.88 100.96,58.1 103.19,55.88
N$20
  Bottom 0.406: IC2.2 16.19,29.84 15.56,29.21 R2.U1
N$21
  Top 0.305: 95.57,58.58 95.57,53.34 arc-90 94.3,54.61 94.3,57.31 arc-90 95.57,58.58
N$22
  Bottom 0.305: IC6.20 77.08,26.59 77.47,26.19 77.47,25.4 C3.1
N$23
  Bottom 0.406: JP1.16 62.21,67.66 Q3.C
N$24
  Bottom 0.406: Q3.B R8.1
N$25
  Bottom 0.406: JP1.15 55.27,66.18 56.04,65.41 R13.1
N$26  (via drill 0.8 pad 1.68)
  Top 0.406: v34.61,33.66 v52.86,33.66
  Bottom 0.305: C17.2 32.13,35.37 R7.3 27.91,33.4 R7.2
  Bottom 0.406: C17.2 33.21,35.37 33.66,34.92 33.66,34.13 34.13,33.66 v34.61,33.66 IC3.7 | R23.1 52.86,31.11 v52.86,33.66
N$27
  Bottom 0.406: IC3.12 45.72,28.57 46.36,29.21 49.7,29.21 R17.1 R16.1
N$28  (via drill 0.8 pad 1.68)
  Top 0.406: v54.93,25.4 v54.93,16.67
  Bottom 0.406: IC1.1 v54.93,25.4 | v54.93,16.67 52.71,14.45 35.72,14.45 32.23,17.93 R22.2
N$29
  Bottom 0.305: R3.2 60.64,38.26 60.64,31.11 61.28,30.48 IC1.12
N$30
  Bottom 0.406: IC3.2 IC3.13 45.72,27.3 46.36,27.94 51.43,27.94 52.71,26.67 C7.2 54.61,27.94 IC1.3
N$31
  Top 0.305: 93.03,58.42 arc90 91.76,57.15 91.76,56.52 arc90 92.39,55.88 arc-90 93.03,55.25 93.03,54.61 arc-90 91.76,53.34
N$32
  Top 0.305: 89.22,55.88 90.33,55.88
N$33
  Bottom 0.406: R24.1 R6.2 38.73,35.56 38.73,32.7 38.42,32.39 IC3.6 35.4,32.39 35.24,32.23 33.81,32.23 33.66,32.39 32.89,32.39 32.7,32.57 C17.1
N$34
  Top 0.305: 85.41,53.34 86.04,58.42 86.68,54.61 87.31,58.42 87.95,53.34
N$35
  Bottom 0.305: R7.1 30.16,36.04 30.8,36.67 33.66,36.67 R24.2
N$36
  Top 0.305: 10.95,53.97 10.95,56.52 | 8.41,64.77 5.87,64.77 | 3.33,64.77 0.79,64.77 0.79,56.52 | 0.79,53.97 0.79,51.44 3.33,51.44 | 3.33,51.44 5.87,51.44 | 8.41,51.44 10.95,51.44 10.95,53.97 | 10.95,53.97 0.79,53.97 | 0.79,53.97 0.79,56.52 | 0.79,56.52 10.95,56.52 | 10.95,56.52 10.95,64.77 8.41,64.77 | 8.41,64.77 8.41,51.44 | 8.41,51.44 5.87,51.44 | 5.87,51.44 5.87,64.77 | 5.87,64.77 3.33,64.77 | 3.33,64.77 3.33,51.44
N$37
  Top 0.254: 19.68,65.88 21.27,64.29 22.23,64.29 | 33.02,64.29 32.38,64.29 | 32.38,65.88 32.38,64.29 | 32.38,64.29 29.84,64.29 | 29.84,65.88 29.84,64.29 | 29.84,64.29 27.31,64.29 | 27.31,65.88 27.31,64.29 | 27.31,64.29 24.76,64.29 | 24.76,65.88 24.76,64.29 | 24.76,64.29 22.23,64.29 | 22.23,64.29 22.23,65.88
N$38
  Top 0.254: 34.93,65.88 34.93,65.25
N$39
  Top 0.254: 37.47,65.09 37.47,65.88
N$40
  Top 0.254: 40,65.56 40,65.88
N$41
  Top 0.254: 42.54,65.09 42.54,65.88
N$42
  pour Top (isolate 1.422): 0,0 107.31,0 107.31,71.12 0,71.12
N$43
  Top 0.254: 50.17,65.88 50.17,64.29 | 50.17,64.29 50.32,64.29 52.71,64.29 | 52.71,65.88 52.71,64.29 | 52.71,64.29 55.25,64.29 | 55.25,65.88 55.25,64.29 | 55.25,64.29 56.36,64.29 57.94,65.88 | 47.78,64.29 50.17,64.29 | 43.97,64.29 45.08,64.29 | 45.08,65.88 45.08,64.29 | 45.08,64.29 47.47,64.29 47.62,64.29 | 47.62,65.88 47.62,64.29 | 50.17,64.29 47.62,64.29
N$44
  pour Bottom (isolate 1.27): 0,0 107.31,0 107.31,71.12 0,71.12
N$45
  Bottom 1.016: IC7.IN 42.07,41.91 D3.C 34.61,41.67 C19.+ C13.1 D2.C
N$46
  cutout Top (isolate 1.27): 105.89,50.32 83.82,50.32 83.82,58.9 68.88,58.88 68.88,63.8 84.14,63.82 84.14,66.2 105.89,66.2
N$47
  cutout Bottom: 73.34,34.92 80.01,34.92 80.01,28.26 73.34,28.26
PB0  (via drill 0.8 pad 1.68)
  Top 0.305: v67.15,27.3 v84.14,27.3
  Bottom 0.305: R5.2 52.24,17.63 54.93,20.32 65.25,20.32 68.42,23.5 68.42,26.04 v67.15,27.3 | v84.14,27.3 86.36,27.3 86.99,27.94 86.99,29.84 86.36,30.48 84.77,30.48 84.3,30 83.19,30 82.87,30.32 82.87,30.96 81.83,31.99 IC6.12
  Bottom 0.406: R5.2 48.56,17.63 Q2.E
PB1  (via drill 0.8 pad 1.68)
  Top 0.305: v85.25,29.21 v85.25,35.72 | v82.87,35.72 v70.01,35.72
  Bottom 0.305: IC6.13 81.84,31.19 82.39,30.64 82.39,30 83.19,29.21 v85.25,29.21 | v85.25,35.72 v82.87,35.72 | v70.01,35.72 69.53,35.72 68.74,36.51 JP2.2
PC0  (via drill 0.8 pad 1.68)
  Top 0.305: v99.38,17.78 v73.98,17.78
  Bottom 0.305: JP1.11 45.11,64.59 45.56,64.14 47.31,64.14 47.78,63.66 49.53,63.66 50.01,63.18 51.91,63.18 52.39,62.71 66.52,62.71 66.99,62.23 101.12,62.23 102.87,60.48 102.87,20 100.65,17.78 v99.38,17.78 | IC6.23 74.68,18.48 v73.98,17.78
PC1  (via drill 0.8 pad 1.68)
  Top 0.305: v97.31,16.51 v71.6,16.51
  Bottom 0.305: JP1.12 47.65,64.59 48.1,64.14 49.85,64.14 50.32,63.66 52.23,63.66 52.71,63.18 66.83,63.18 67.31,62.71 101.44,62.71 103.35,60.8 103.35,19.21 100.65,16.51 v97.31,16.51 | v71.6,16.51 71.6,17.3 73.88,19.58 IC6.24
PC2  (via drill 0.8 pad 1.68)
  Top 0.305: v99.38,15.24 v73.98,15.24
  Bottom 0.305: JP1.13 50.19,64.59 50.64,64.14 52.55,64.14 53.02,63.66 67.15,63.66 67.63,63.18 101.76,63.18 103.82,61.12 103.82,18.41 100.65,15.24 v99.38,15.24 | v73.98,15.24 70.8,15.24 70.33,15.72 70.33,17.3 71.44,18.41 71.44,28.57 71.65,28.79 IC6.25
PC3  (via drill 0.8 pad 1.68)
  Top 0.305: v97.31,13.97 v72.07,13.97
  Bottom 0.305: JP1.14 52.73,64.75 53.34,64.14 67.47,64.14 67.94,63.66 102.08,63.66 104.3,61.44 104.3,17.62 100.65,13.97 v97.31,13.97 | v72.07,13.97 70.8,13.97 69.69,15.08 69.69,17.46 70.96,18.73 70.96,28.89 71.66,29.59 IC6.26
PC4  (via drill 0.8 pad 1.68)
  Top 0.305: v99.38,20.32 v68.9,20.32
  Bottom 0.305: JP1.4 27.33,64.59 27.78,64.14 32.07,64.14 32.54,63.66 44.45,63.66 44.93,63.18 46.67,63.18 47.15,62.71 48.9,62.71 49.37,62.23 51.28,62.23 51.75,61.75 65.88,61.75 66.36,61.28 100.49,61.28 101.92,59.85 101.92,21.59 100.65,20.32 v99.38,20.32 | v68.9,20.32 70.49,21.91 70.49,29.21 71.67,30.39 IC6.27
PC5  (via drill 0.8 pad 1.68)
  Top 0.305: v67.31,19.05 v97.47,19.05
  Bottom 0.305: JP1.6 32.41,64.59 32.86,64.14 44.77,64.14 45.24,63.66 46.99,63.66 47.47,63.18 49.21,63.18 49.69,62.71 51.59,62.71 52.07,62.23 66.2,62.23 66.68,61.75 100.81,61.75 102.39,60.17 102.39,20.8 100.65,19.05 v97.47,19.05 | v67.31,19.05 67.31,20.48 70.01,23.18 70.01,29.53 71.67,31.19 IC6.28
PD3  (via drill 0.8 pad 1.68)
  Top 0.305: v73.18,42.55 v105.73,42.55
  Bottom 0.305: R8.2 67.63,64.77 68.26,64.14 102.39,64.14 104.77,61.75 104.77,43.5 v105.73,42.55 | IC6.1 73.88,39.15 73.18,39.85 v73.18,42.55
PD4  (via drill 0.8 pad 1.68)
  Top 0.305: v74.45,40.64 v85.25,40.64
  Bottom 0.254: 74.68,40.39 74.68,40.42 v74.45,40.64
  Bottom 0.305: IC6.2 74.68,40.39 | v85.25,40.64 85.25,37.78 85.88,37.15 95.41,37.15 98.11,34.45 98.11,21.91 86.84,10.64 84.14,10.64 83.5,10 R19.1 81.12,8.73 80.72,8.33 S1.2
  Bottom 0.61: S1.2 S1.1
PD5
  Bottom 0.305: IC6.9 95.31,34.39 97.63,32.07 97.63,22.23 86.52,11.11 83.82,11.11 83.34,10.64 70.96,10.64 70.17,9.84 R18.1 67.15,8.73 66.75,8.33 S2.2
  Bottom 0.61: S2.2 S2.1
PD6
  Bottom 0.305: IC6.10 95.31,33.59 97.16,31.75 97.16,22.54 86.2,11.59 83.5,11.59 83.03,11.11 70.64,11.11 70.17,10.64 56.99,10.64 56.2,9.84 R20.1 53.18,8.73 52.78,8.33 S3.2
  Bottom 0.61: S3.1 S3.2
PD7
  Bottom 0.305: IC6.11 95.32,32.79 96.68,31.43 96.68,22.86 85.88,12.06 83.19,12.06 82.71,11.59 70.33,11.59 69.85,11.11 56.67,11.11 56.2,10.64 43.02,10.64 42.23,9.84 R21.1 39.21,8.73 38.81,8.33 S4.2
  Bottom 0.61: S4.1 S4.2
RESET  (via drill 0.8 pad 1.68)
  Top 0.305: v83.98,31.43 v70.01,31.43
  Bottom 0.305: C6.2 R1.1 68.58,31.59 68.74,31.43 v70.01,31.43 70.57,31.99 IC6.29 | SV1.5 93.5,31.75 93.03,32.23 84.77,32.23 v83.98,31.43
SCK
  Bottom 0.305: IC6.17 79.48,23.87 80.49,22.86 93.82,22.86 95.25,24.29 95.25,26.67 SV1.3
VCC  (via drill 0.8 pad 1.68)
  Top 0.406: v19.37,21.59 v19.37,39.37
  Bottom 0.406: v19.37,39.37 19.37,41.67 D2.A | R15.2 23.03,17.93 v19.37,21.59
  Bottom 0.813: 5.08,38.42 X2.1
  Bottom 1.016: R2.I2 18.1,41.91 D2.A
  Bottom 2.184: R2.I2 6.03,39.37 5.08,38.42
(copper drawn outside any net)
  shapes: Bottom circle x4

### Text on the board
Top: Februar 2013 | Output | Input | Belegung | Display | 1 | 16 | designed by H.Stockhoff | 4 | 3 | 2 | 1 | + | - | - | + | INPUT | 1 | +In | EXT | -In | ICSP | -Out | 1 | +Out | OUTPUT | 4
Bottom: <C> 2013 | DS-W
